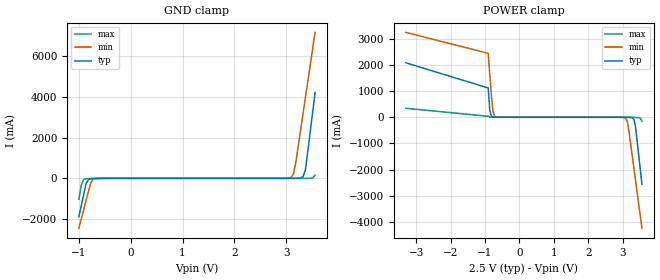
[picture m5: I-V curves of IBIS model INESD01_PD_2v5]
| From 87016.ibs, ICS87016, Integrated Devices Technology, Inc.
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[Model] INESD01_PD_2v5
Model_type   Input
Polarity   Non-Inverting
Vinl = 0.8V
Vinh = 2.0V
|   typ   min   max
C_comp   2pF   1.5pF   2.5pF
|   typ   min   max
[Voltage range]  2.5V   2.375V   2.625V
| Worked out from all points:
|   GND clamp passes 1 mA (typ) near -0.55 V on its own axis
|   POWER clamp passes 1 mA (typ) near -0.68 V on its own axis
[GND_clamp]
|Voltage I(typ)   I(min)   I(max)
-1V       -1.886A    -2.451A    -1.028A
-953.5mV  -1.338A    -1.994A    -328mA
-907mV    -789.6mA   -1.537A    -53.04mA
-860.5mV  -251.4mA   -1.081A    -21.51mA
-767.5mV  -17.28mA   -198.8mA   -10.01mA
-674.5mV  -5.28mA    -15.38mA   -3.684mA
3.092V    224.5uA    49.06mA    51.52uA
3.139V    500.8uA    208.3mA    52.98uA
3.185V    1.252mA    774.6mA    56.66uA
3.325V    81.55mA    3.177A     200uA
3.371V    416.9mA    3.978A     464.6uA
3.557V    4.225A     7.185A     159.2mA
[POWER_clamp]
|Voltage   I(typ)   I(min)   I(max)
-3.3V     2.083A     3.246A     343.1mA
-907mV    1.122A     2.445A     37.78mA
-860.5mV  267.5mA    1.644A     5.973mA
-814mV    47.03mA    844mA      1.727mA
-767.5mV  9.66mA     215.3mA    677uA
-674.5mV  960.6uA    12.66mA    131.4uA
3.092V    -1.849mA   -49.09mA   -51.51uA
3.139V    -3.491mA   -186mA     -159.7uA
3.325V    -84.03mA   -1.955A    -5.102mA
3.371V    -365.4mA   -2.411A    -8.31mA
3.51V     -2.01A     -3.782A    -35.44mA
3.557V    -2.558A    -4.239A    -152.3mA
